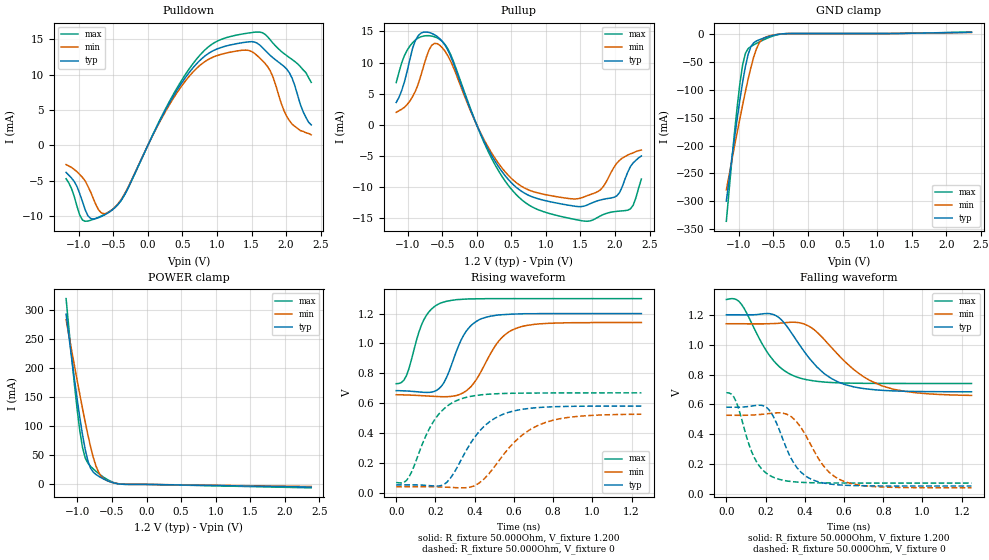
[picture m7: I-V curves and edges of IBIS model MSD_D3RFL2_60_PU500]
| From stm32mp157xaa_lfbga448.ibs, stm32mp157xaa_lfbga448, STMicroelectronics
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[Model] MSD_D3RFL2_60_PU500
Model_type   I/O
C_comp 2.422pF   2.336pF   2.548pF
Vinh = 820.000mV
Vinl = 380.000mV
Vmeas = 600.000mV
Vref = 600.000mV
[Model Spec]
Vinh   820.000mV   790.000mV   870.000mV
Vinl   380.000mV   350.000mV   430.000mV
Vmeas   600.000mV   570.000mV   650.000mV
Vref   600.000mV   570.000mV   650.000mV
[Temperature Range]   25.000   125.000   -40.000
[Voltage Range]   1.200V   1.140V   1.300V
[GND Clamp Reference]   0.00V   0.00V   0.00V
[Pulldown Reference]   0.00V   0.00V   0.00V
[POWER Clamp Reference]   1.200V   1.140V   1.300V
[Pullup Reference]   1.200V   1.140V   1.300V
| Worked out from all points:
|   slope of the pulldown table from 0 to 0.18 V, typ, clamps not added: 50.1 ohm
|   slope of the pullup table from 0 to 0.18 V, typ, clamps not added: 42.9 ohm
|   GND clamp passes 1 mA (typ) near -0.40 V on its own axis
|   POWER clamp passes 1 mA (typ) near -0.41 V on its own axis
|   rising waveform, R_fixture 50.000Ohm, V_fixture 1.200: 20-80 % time 105ps typ, 136ps min, 85.6ps max; typ from 0.685 V to 1.2 V
|   rising waveform, R_fixture 50.000Ohm, V_fixture 0: 20-80 % time 170ps typ, 211ps min, 139ps max; typ from 0.054 V to 0.582 V
|   falling waveform, R_fixture 50.000Ohm, V_fixture 1.200: 20-80 % time 197ps typ, 247ps min, 158ps max; typ from 1.2 V to 0.685 V
|   falling waveform, R_fixture 50.000Ohm, V_fixture 0: 20-80 % time 116ps typ, 143ps min, 98.7ps max; typ from 0.582 V to 0.054 V
[GND Clamp]
-1.182V   -299.2mA   -279.2mA   -335.4mA
-1.064V   -187mA     -201.4mA   -177mA
-984.9mV  -117.5mA   -151.3mA   -88.22mA
-945.5mV  -86.23mA   -127mA     -55.43mA
-906.1mV  -58.85mA   -103.7mA   -35.31mA
-866.7mV  -37.36mA   -81.45mA   -26.92mA
-827.3mV  -23.56mA   -60.91mA   -23.14mA
-748.5mV  -13.42mA   -27.95mA   -17.73mA
-709.1mV  -11.25mA   -17.35mA   -15.24mA
-630.3mV  -7.747mA   -7.41mA    -10.55mA
-472.7mV  -2.393mA   -2.09mA    -3.114mA
2.364V    2.273mA    1.921mA    2.674mA
[Power Clamp]
-1.164V   292.3mA    282.6mA    319mA
-1.085V   218.5mA    230.8mA    219.8mA
-1.006V   148.3mA    180mA      130.9mA
-966.7mV  115.8mA    155.2mA    93.11mA
-927.3mV  86mA       130.8mA    63.78mA
-887.9mV  60.28mA    107.3mA    45.68mA
-809.1mV  27.72mA    64.28mA    30.98mA
-730.3mV  16.96mA    31.12mA    22.29mA
-690.9mV  13.87mA    20.29mA    18.43mA
-572.7mV  6.606mA    6.547mA    8.709mA
-336.4mV  197.1uA    373.8uA    219.2uA
2.382V    -4.548mA   -3.619mA   -5.899mA
[Pulldown]
-1.182V   -3.8mA     -2.7mA     -4.7mA
-945.5mV  -7.91mA    -4.5mA     -10.51mA
-827.3mV  -10.31mA   -6.57mA    -10.56mA
-669.7mV  -10.01mA   -9.53mA    -9.94mA
-551.5mV  -9.372mA   -9.338mA   -9.3mA
-315.1mV  -6.567mA   -6.465mA   -6.608mA
551.5mV   9.678mA    9.198mA    10.13mA
906.1mV   13.16mA    12.3mA     14.14mA
1.261V    14.32mA    13.29mA    15.53mA
1.733V    13.06mA    11.12mA    15.34mA
2.009V    10.78mA    4.11mA     12.69mA
2.364V    2.9mA      1.5mA      8.9mA
[Pullup]
-1.164V   3.6mA      2.005mA    6.785mA
-1.045V   6.9mA      2.809mA    11.11mA
-887.9mV  13.51mA    5.376mA    13.62mA
-690.9mV  14.84mA    11.99mA    14.32mA
-454.5mV  12.73mA    11.77mA    12.85mA
175.8mV   -4.107mA   -3.772mA   -4.491mA
687.9mV   -10.94mA   -10.12mA   -12.36mA
1.476V    -13.13mA   -11.84mA   -15.31mA
1.791V    -12.06mA   -10.42mA   -14.61mA
1.988V    -11.63mA   -6.784mA   -13.94mA
2.224V    -6.7mA     -4.648mA   -13.49mA
2.382V    -5mA       -4.048mA   -8.7mA
[Ramp]
R_load=50.000Ohm
dV/dt_r   312.813mV/138.000ps  290.544mV/174.500ps  346.668mV/112.500ps
dV/dt_f   312.843mV/157.500ps  290.541mV/197.500ps  346.668mV/129.000ps
[Rising waveform]
R_fixture=50.000Ohm
V_fixture=1.200
V_fixture_min=1.140
V_fixture_max=1.300
0s        684.8mV    657.3mV    731.2mV
52ps      682.5mV    655.8mV    784.7mV
115ps     676.2mV    652.2mV    1.073V
141ps     673.4mV    650.3mV    1.159V
230ps     713.5mV    644.3mV    1.272V
345ps     1.058V     672.9mV    1.296V
435ps     1.166V     818.5mV    1.299V
524ps     1.191V     1.018V     1.3V
626ps     1.198V     1.108V     1.3V
1.25ns    1.2V       1.14V      1.3V
[Rising waveform]
R_fixture=50.000Ohm
V_fixture=0
0s        54.44mV    42.34mV    70.59mV
64ps      54.76mV    42.59mV    105.3mV
166ps     50.22mV    42.43mV    423.2mV
230ps     50.76mV    40.74mV    546.3mV
320ps     194.6mV    35.31mV    624.8mV
435ps     428.6mV    79.84mV    657.1mV
575ps     540.5mV    301.9mV    666.7mV
677ps     565.7mV    419.6mV    668.4mV
805ps     577.2mV    488.8mV    669.2mV
1.25ns    581.5mV    527mV      670mV
[Falling waveform]
R_fixture=50.000Ohm
V_fixture=1.200
V_fixture_min=1.140
V_fixture_max=1.300
0s        1.2V       1.14V      1.302V
77ps      1.199V     1.14V      1.27V
243ps     1.2V       1.141V     889.3mV
358ps     1.028V     1.149V     784.1mV
422ps     910.6mV    1.123V     762.9mV
498ps     807.6mV    1.036V     750.1mV
613ps     730.1mV    876.5mV    743mV
728ps     702mV      763.2mV    741.1mV
843ps     691.2mV    705.2mV    740.5mV
1.25ns    684.8mV    660.6mV    740.3mV
[Falling waveform]
R_fixture=50.000Ohm
V_fixture=0
0s        581.5mV    527.7mV    678.4mV
52ps      581.3mV    527.4mV    612.5mV
154ps     593.7mV    530.9mV    216.7mV
205ps     580.4mV    537.4mV    139.2mV
256ps     474.8mV    543.7mV    104.7mV
358ps     180.9mV    484.1mV    81.2mV
460ps     86.38mV    260.1mV    75.83mV
549ps     64.86mV    120.5mV    74.77mV
652ps     57.41mV    66.53mV    74.42mV
1.25ns    54.3mV     42.34mV    74.24mV
